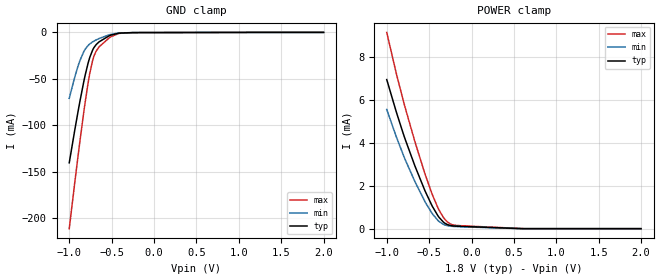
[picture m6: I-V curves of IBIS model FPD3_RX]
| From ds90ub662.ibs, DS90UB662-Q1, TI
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|   FPD3_RX Model
[Model]   FPD3_RX
Model_type   Input
Vinl = 0.54
Vinh = 1.26
|   typ   min   max
C_comp   0.938pF   0.681pF   1.119pF
[Voltage Range]   1.8   1.71   1.89
[Temperature Range]   27   105   -40
[Power Clamp Reference]   1.8   1.71   1.89
[GND Clamp Reference]   0   0   0
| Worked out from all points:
|   GND clamp passes 1 mA (typ) near -0.42 V on its own axis
|   POWER clamp passes 1 mA (typ) near -0.46 V on its own axis
[GND Clamp]
|   Voltage   I(typ)   I(min)   I(max)
-1V       -140.4mA   -70.99mA   -211.3mA
-934mV    -104.8mA   -47.84mA   -161.1mA
-874mV    -74.21mA   -30.36mA   -117.2mA
-811mV    -45.64mA   -17.98mA   -74.44mA
-757mV    -26.72mA   -12.35mA   -43.75mA
-721mV    -18.46mA   -10.03mA   -29.2mA
-682mV    -13.12mA   -8.077mA   -20.08mA
-646mV    -10.06mA   -6.531mA   -15.43mA
-532mV    -3.846mA   -2.685mA   -6.148mA
-418mV    -868uA     -725.6uA   -1.195mA
-250mV    -225.5uA   -189.6uA   -282.9uA
2V        0A         0A         0A
[POWER Clamp]
|   Voltage   I(typ)   I(min)   I(max)
-1V       6.95mA     5.555mA    9.149mA
-892mV    5.505mA    4.336mA    7.316mA
-805mV    4.427mA    3.438mA    5.966mA
-670mV    2.948mA    2.214mA    4.088mA
-553mV    1.805mA    1.288mA    2.602mA
-469mV    1.095mA    735.1uA    1.658mA
-397mV    605.9uA    385.2uA    980.7uA
-331mV    303.1uA    200.4uA    519.7uA
-283mV    187.4uA    138.7uA    306.4uA
-172mV    116uA      95.44uA    149.8uA
626mV     0A         0A         397.9nA
2V        0A         0A         0A
